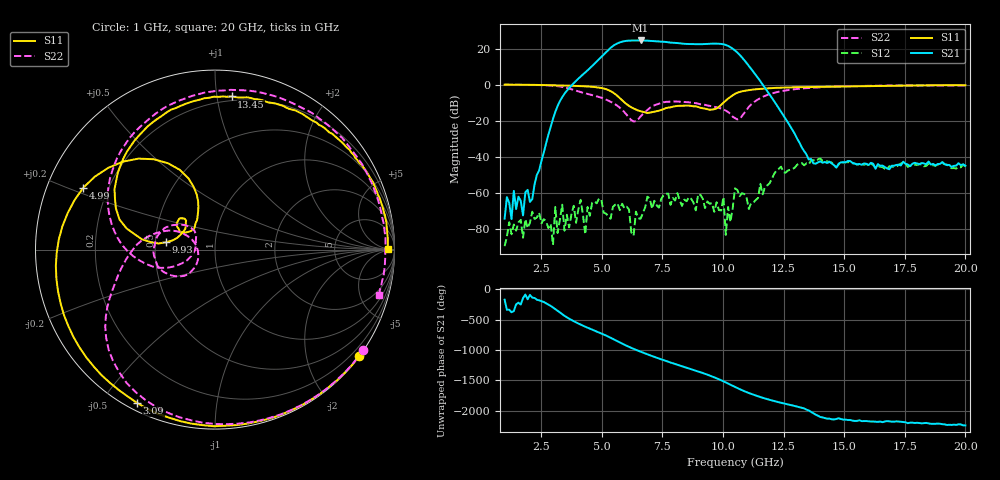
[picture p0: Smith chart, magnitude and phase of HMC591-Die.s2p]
! Analog Devices, Inc.
! Device:  HMC591-Die
! Description:	GaAs PHEMT MMIC 2 WATT POWER AMPLIFIER, 6 - 10 GHz
! Conditions:	Vdd = 7.0 V
!  Vgg = -0.32 V
!  Iddq = 1335 mA
!  Pin = -31 dBm
!  Operating Temperature = +25C
! Engineering Evaluation unit (SN3) measured on PCB
! Measurements are referenced to PCB coaxial connectors
! Freq(GHz)	S11a(dB)	S11p(deg)	S21a(dB)	S21p(deg)	S12a(dB)	S12p(deg)	S22a(dB)	S22p(deg)
# GHz S DB R 50
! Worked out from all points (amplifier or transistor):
!   201 points, 1 GHz to 20 GHz, reference 50 ohm
!   highest |S21| = 24.5 dB at 6.605 GHz (marker M1)
!   |S21| within 3 dB of that: 5.474 GHz to 10.21 GHz (4.739 GHz wide, 60.4 % of centre)
!   unconditionally stable (mu >= 1): start of sweep to end of sweep
!   at 4.135 GHz: K = 48.28, MAG = 14.3 dB, |S12| = -63.8 dB
!   at 10.5 GHz: K = 28.46, MAG = 20.6 dB, |S12| = -57.4 dB
!   at 20 GHz: K = 125.29, MAG = -23.7 dB, |S12| = -45.5 dB
!   S11 on the Smith chart (normalised r, x): 1 GHz: 0.01, -3.04; 3.09 GHz: 0.03, -0.61; 4.99 GHz: 0.11, +0.22; 9.93 GHz: 0.57, +0.05; 13.45 GHz: 0.17, +1.10; 20 GHz: 52, +6
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1  -0.02 -36.4  -74.24 -172.1  -89.44 -104.5  -0.02 -34.2
3.09  -0.37 -117.0  -15.08 31.9  -67.74 90.9  -0.69 -114.7
4.23  -0.87 -165.2  5.64 119.2  -72.01 178.3  -4.48 -160.3
4.99  -1.82 154.9  15.42 -9.1  -63.90 76.0  -7.23 176.2
5.275  -2.98 136.3  19.23 -60.7  -72.86 132.2  -8.81 166.9
5.56  -5.23 118.5  22.22 -118.6  -66.48 90.5  -10.88 158.4
5.94  -9.79 108.3  24.08 165.3  -68.50 97.2  -15.23 153.6
6.225  -12.55 113.4  24.43 112.9  -81.83 78.3  -19.66 170.3
6.605  -14.67 125.1  24.47 50.7  -74.25 122.3  -17.63 -141.7
6.985  -15.50 141.0  24.31 -7.7  -63.01 113.4  -12.90 -139.7
7.365  -14.42 150.1  23.97 -62.6  -68.10 126.8  -10.55 -152.8
7.65  -12.98 152.3  23.65 -102.8  -60.39 95.2  -9.54 -164.5
8.125  -11.77 145.7  23.04 -165.6  -60.03 78.1  -9.36 178.4
8.885  -12.00 135.8  22.49 96.4  -69.57 71.5  -10.24 157.4
9.455  -13.91 145.4  22.68 17.4  -65.93 80.3  -11.77 147.9
9.93  -11.19 171.5  22.54 -61.2  -69.68 97.2  -13.20 141.2
10.5  -5.07 162.5  18.94 -171.1  -57.42 160.2  -18.52 154.3
11.26  -2.69 132.0  7.07 61.4  -65.30 127.9  -9.93 -161.4
13.445  -1.33 83.8  -38.63 175.3  -43.61 75.3  -1.93 121.7
13.73  -1.30 79.8  -43.57 113.0  -41.77 59.7  -1.66 113.8
16.865  -0.65 38.8  -46.87 -17.8  -45.18 -24.8  -0.51 41.2
20  -0.33 0.3  -44.88 -86.2  -45.53 -95.7  -0.47 -15.5
